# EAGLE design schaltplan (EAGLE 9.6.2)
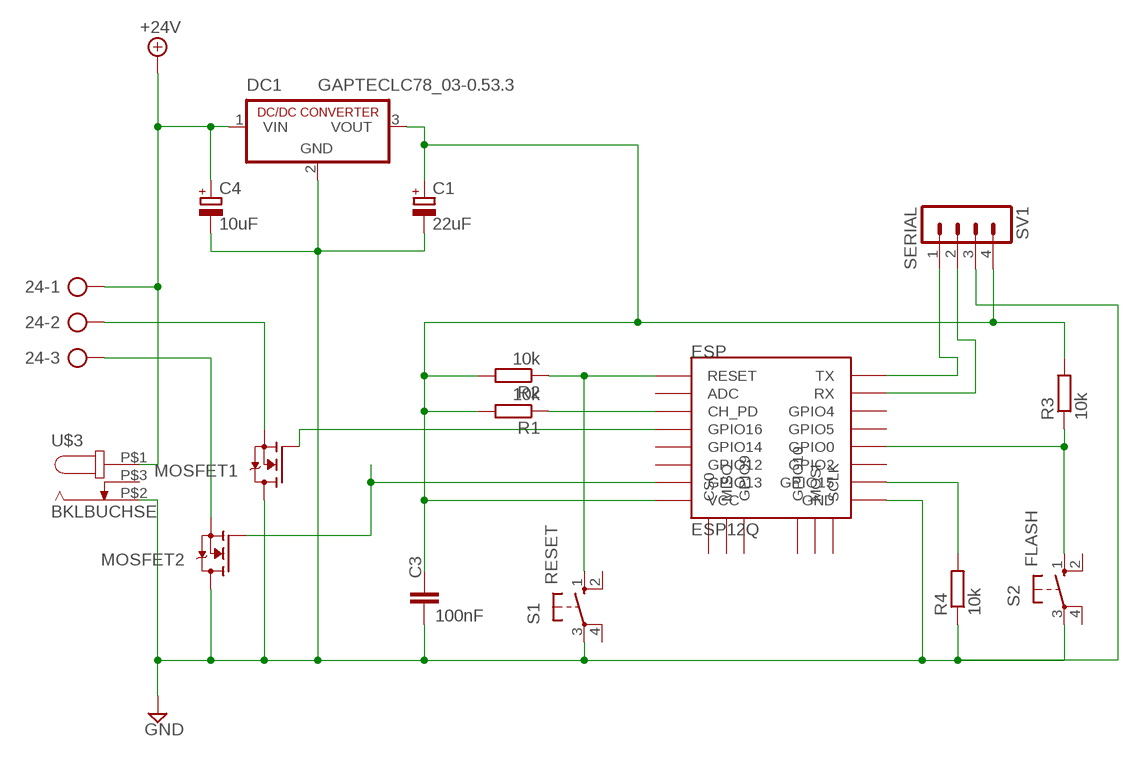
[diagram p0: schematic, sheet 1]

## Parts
24  24/CW/WW  AK500/3  [AK500/3]
C1  22uF  CPOL-EUE1.8-4  [E1,8-4]
C3  100nF  C-EU050-030X075  [C050-030X075]
C4  10uF  CPOL-EUE2.5-6  [E2,5-6]
DC1  GAPTECLC78_03-0.53.3  [SIP3]
ESP  ESP12Q  [ESP12Q]
MOSFET1  IRLZ24N  [TO220ABS]
MOSFET2  IRLZ24N  [TO220ABS]
R1  10k  R-EU_0207/7  [0207/7]
R2  10k  R-EU_0207/7  [0207/7]
R3  10k  R-EU_0207/7  [0207/7]
R4  10k  R-EU_0207/7  [0207/7]
S1  RESET  10-XX  [B3F-10XX]
S2  FLASH  10-XX  [B3F-10XX]
SV1  SERIAL  MA04-1  [MA04-1]
U$3  BKLBUCHSE  [DCJACK]

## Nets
3,3V: C1.+ C3.1 DC1.3(VOUT) ESP.VCC R1.2 R2.2 R3.2 SV1.4
+24V: 24.1 C4.+ DC1.1(VIN) U$3.P$1
CHPD: ESP.CH_PD R1.1
FLS: ESP.GPIO0 R3.1 S2.1(S)
GND: C1.- C3.2 C4.- DC1.2(GND) ESP.GND MOSFET1.C(D) MOSFET2.C(D) R4.1 S1.3(P) S2.3(P) SV1.3 U$3.P$2
GNDX: ESP.GPIO15 R4.2
MS1: 24.2 MOSFET1.A2(S)
MS1G: ESP.GPIO16 MOSFET1.A1(G)
MS2: 24.3 MOSFET2.A2(S)
MS2G: ESP.GPIO13 MOSFET2.A1(G)
RST: ESP.RESET R2.1 S1.1(S)
RX: ESP.RX SV1.2
TX: ESP.TX SV1.1
Unconnected: ESP.ADC ESP.CS0 ESP.GPIO2 ESP.GPIO4 ESP.GPIO5 ESP.GPIO9 ESP.GPIO10 ESP.GPIO12 ESP.GPIO14 ESP.MISO ESP.MOSI ESP.SCLK S1.2(S1) S1.4(P1) S2.2(S1) S2.4(P1) U$3.P$3

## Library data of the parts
24 = con-ptr500:AK500/3: CONNECTOR; OC_FARNELL: unknown; OC_NEWARK: unknown
C1 C4 = rcl:CPOL-EU: POLARIZED CAPACITOR, European symbol; SPICEPREFIX: C
C3 = resistor:C-EU: CAPACITOR, European symbol
DC1 = cct:GAPTECLC78_03-0.5: Gaptec DC/DC-Converter 0,5 AMP SIP3 Single Output Auf 3.3V Source: Data sheet
ESP = esp826612q:ESP12Q: ESP8266 Wifi module 12-Q
MOSFET1 MOSFET2 = cct:IRLZ24N: Mosfet IRLZ24N
R1-R4 = rcl:R-EU_: RESISTOR, European symbol; SPICEPREFIX: R
S1 S2 = switch-omron:10-XX: OMRON SWITCH; MPN: B3F-1000; OC_FARNELL: 176432; OC_NEWARK: 36M3542
SV1 = con-lstb:MA04-1: PIN HEADER; OC_FARNELL: unknown; OC_NEWARK: unknown
U$3 = cct:BKLBUCHSE

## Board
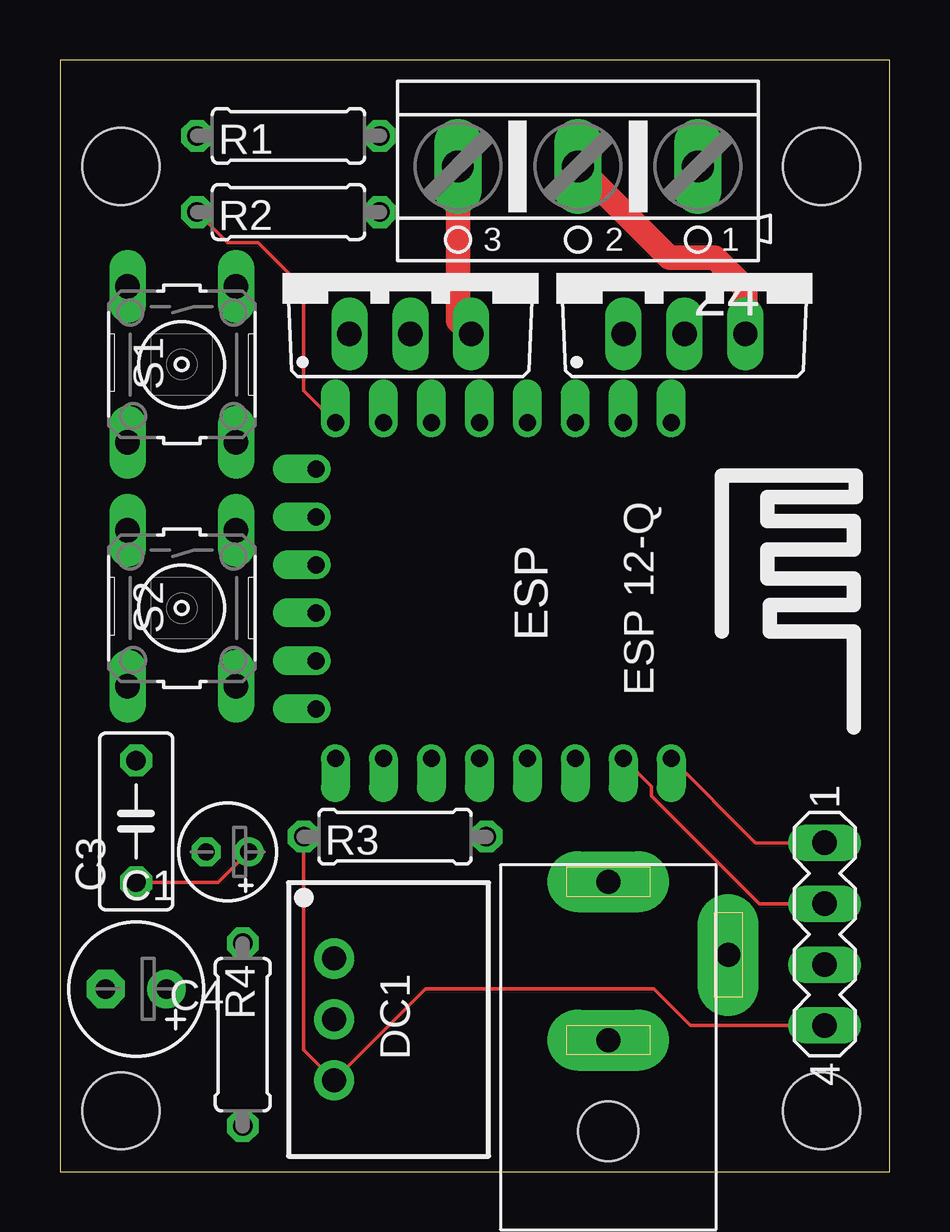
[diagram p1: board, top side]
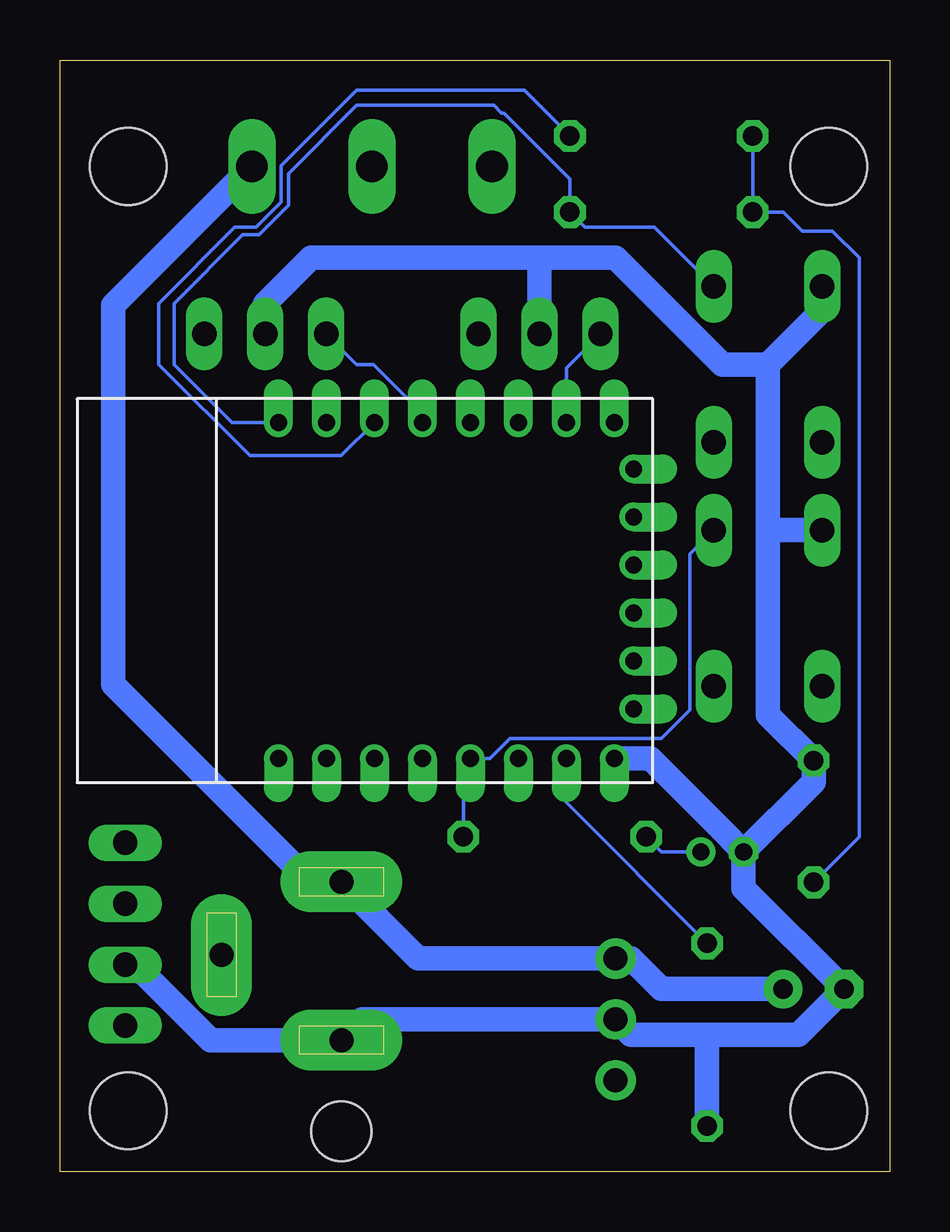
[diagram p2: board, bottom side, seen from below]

Size 34.59 x 46.34 mm. Coordinates in mm from the lower left corner, seen from the top.
Outline: 0,0 34.59,0 34.59,46.34 0,46.34 0,0
Copper layers (1*16): Top 0.035mm / dielectric 1.5mm / Bottom 0.035mm
Design rules "default": minimum track width 6mil, minimum drill 0.35mm, track to track 6mil, track to pad 6mil, pad to pad 6mil, via to via 6mil, smd to smd 6mil, copper to edge 40mil, drill to drill 6mil, minimum pad ring 10mil, minimum via ring 8mil, stop-mask expansion 4mil, vias tented up to drill 0mil, thermal gap 10mil
Holes 3.2 mm at 31.75,2.54 2.54,2.54 31.75,41.91 2.54,41.91

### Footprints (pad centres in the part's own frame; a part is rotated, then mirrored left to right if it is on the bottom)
AK500/3 = drill 1.321 long: 1 -5.004,0; 2 0,0; 3 5.004,0
E1,8-4 = drill 0.711 pad 1.168: + -0.889,0 | drill 0.711 pad 1.168 octagon: - 0.889,0
C050-030X075 = drill 0.813 octagon: 1 -2.54,0; 2 2.54,0
E2,5-6 = drill 0.813 pad 1.6: + -1.27,0 | drill 0.813 pad 1.6 octagon: - 1.27,0
SIP3 = drill 1 pad 1.676: 1 -2.54,0; 2 0,0; 3 2.54,0
ESP12Q = drill 0.7 offset: ADC -7.1,3.8; CH_PD -7.1,1.8; CS0 -5.165,-9.005; GND 6.9,-8.2; GPIO0 6.9,-2.2; GPIO2 6.9,-4.2; GPIO4 6.9,1.8; GPIO5 6.9,-0.2; GPIO9 -1.165,-9.005; GPIO10 0.835,-9.005; GPIO12 -7.1,-4.2; GPIO13 -7.1,-6.2; GPIO14 -7.1,-2.2; GPIO15 6.9,-6.2; GPIO16 -7.1,-0.2; MISO -3.165,-9.005; MOSI 2.835,-9.005; RESET -7.1,5.8; RX 6.9,3.8; SCLK 4.835,-9.005; TX 6.9,5.8; VCC -7.1,-8.2
TO220ABS = drill 1.016 long: A1 -2.54,-2.54; A2 2.54,-2.54; C 0,-2.54
0207/7 = drill 0.813 octagon: 1 -3.81,0; 2 3.81,0
B3F-10XX = drill 1.016 long: 1 -3.251,2.261; 2 3.251,2.261; 3 -3.251,-2.261; 4 3.251,-2.261
MA04-1 = drill 1.016 long: 1 -3.81,0; 2 -1.27,0; 3 1.27,0; 4 3.81,0
DCJACK = drill 1 pad 2.54 long: P$1 0,14.5; P$2 0,7.9; P$3 5,11.45 | hole 2.5: 0,4.1

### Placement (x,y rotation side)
24  21.59,41.91 180 top
C1  6.98,13.33 180 top
C3  3.18,14.6 90 top
C4  3.18,7.62 180 top
DC1  11.43,6.35 270 top
ESP  19.69,24.13 270 top
MOSFET1  26.03,37.47 0 top
MOSFET2  14.6,37.47 0 top
R1  9.52,43.18 180 top
R2  9.52,40.01 180 top
R3  13.97,13.97 180 top
R4  7.62,5.71 90 top
S1  5.08,33.66 270 top
S2  5.08,23.5 270 top
SV1  31.88,9.91 270 top
U$3  22.86,-2.41 0 top

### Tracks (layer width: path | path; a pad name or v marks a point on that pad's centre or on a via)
3,3V
  Top 0.152: SV1.4 26.29,6.1 24.77,7.62 15.24,7.62 DC1.3 10.16,5.08 R3.2 | C1.+ 6.6,12.06 C3.1 | R2.2 6.98,38.73 8.25,38.73 10.16,36.83 10.16,32.55 ESP.VCC
  Bottom 0.152: R3.2 9.52,13.33 C1.+ | C3.1 1.27,13.97 1.27,38.1 2.39,39.22 3.66,39.22 4.44,40.01 R2.2 R1.2
+24V
  Bottom 1.016: 24.1 32.38,36.12 32.38,20.32 24.15,12.09 U$3.P$1 19.66,8.89 DC1.1 10.79,8.89 9.52,7.62 C4.+
CHPD
  Bottom 0.152: R1.1 15.24,45.09 22.23,45.09 25.38,41.94 25.38,40.41 26.42,39.37 27.3,39.37 30.48,36.2 30.48,33.66 26.67,29.85 22.87,29.85 ESP.CH_PD
FLS
  Bottom 0.152: S2.1 8.33,25.76 8.33,19.26 9.53,18.06 15.83,18.06 16.66,17.23 ESP.GPIO0 17.78,16.93 R3.1
GND
  Bottom 1.016: SV1.3 31.46,8.64 28.31,5.49 U$3.P$2 22,6.35 DC1.2 10.79,5.71 7.62,5.71 | 7.62,5.71 3.81,5.71 C4.- 6.1,11.81 C1.- | R4.1 7.62,5.71 | C1.- 3.18,16.26 C3.2 5.08,19.05 5.08,26.67 | C1.- 6.6,13.84 6.6,13.86 9.97,17.23 ESP.GND | 5.08,26.67 5.08,33.66 | S2.3 5,26.75 5.08,26.67 | 5.08,33.66 6.98,33.66 11.43,38.1 14.6,38.1 | 14.6,38.1 24.13,38.1 26.03,36.2 MOSFET1.C | S1.3 2.82,35.92 5.08,33.66 | 14.6,38.1 MOSFET2.C
GNDX
  Bottom 0.152: R4.2 13.48,15.39 ESP.GPIO15
MS1
  Top 1.016: 24.2 25.4,38.1 27.3,38.1 28.58,36.83 MOSFET1.A2
MS1G
  Bottom 0.152: MOSFET1.A1 22.23,33.66 21.52,33.66 19.48,31.62 ESP.GPIO16
MS2
  Top 1.016: 16.59,40.72 24.3 16.59,35.48 MOSFET2.A2
MS2G
  Bottom 0.152: MOSFET2.A1 13.48,33.51 ESP.GPIO13
RST
  Bottom 0.152: S1.1 9.8,39.37 12.7,39.37 R2.1 13.34,41.37 16.08,44.12 16.18,44.12 16.51,44.45 22.23,44.45 25.07,41.61 25.07,40.29 26.29,39.06 26.98,39.06 29.84,36.2 29.84,33.66 27.42,31.23 ESP.RESET
RX
  Top 0.152: ESP.RX 24.65,16.06 24.65,15.68 29.15,11.18 SV1.2
TX
  Top 0.152: ESP.TX 29,13.72 SV1.1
